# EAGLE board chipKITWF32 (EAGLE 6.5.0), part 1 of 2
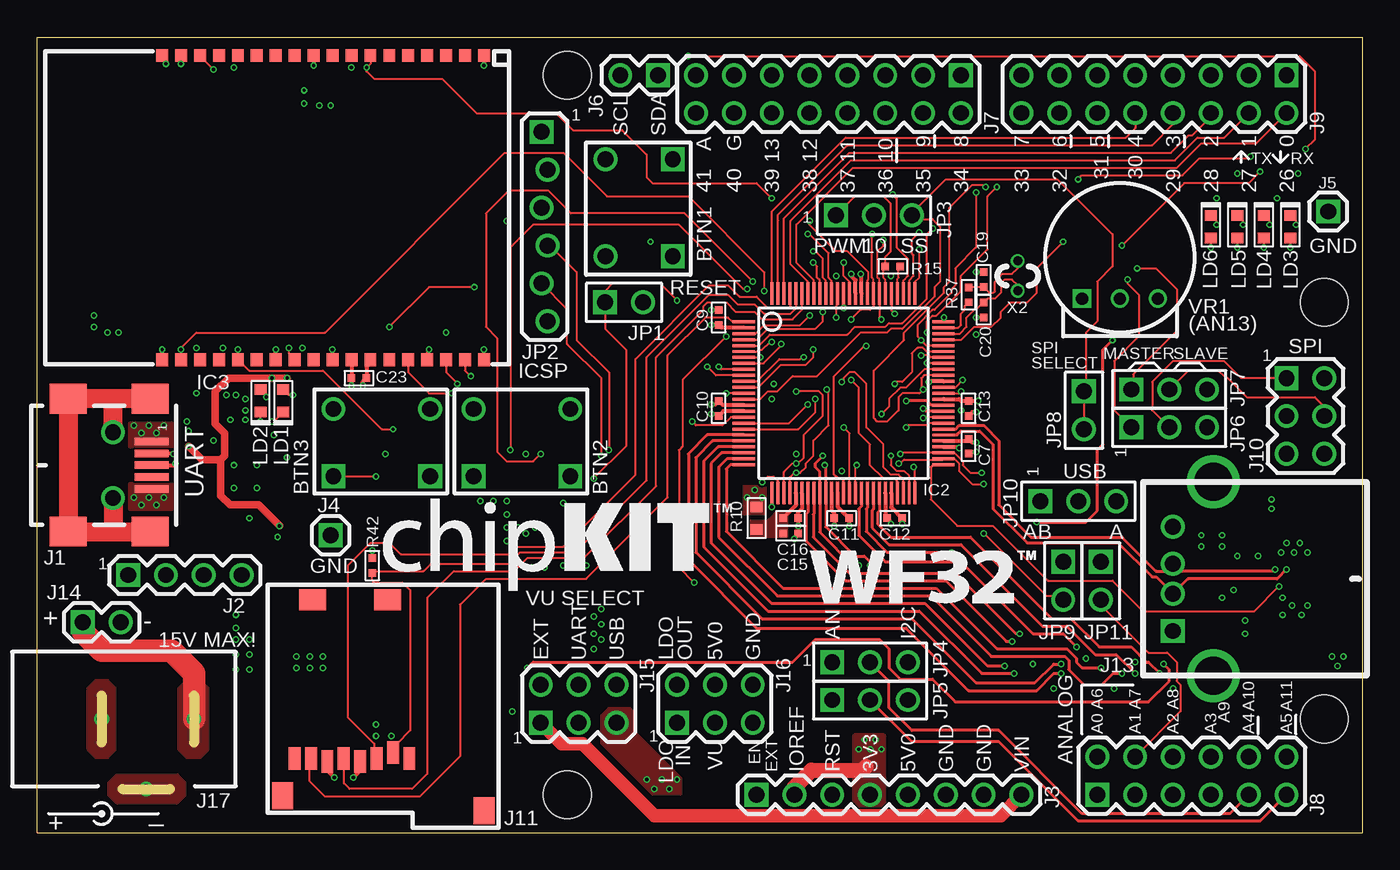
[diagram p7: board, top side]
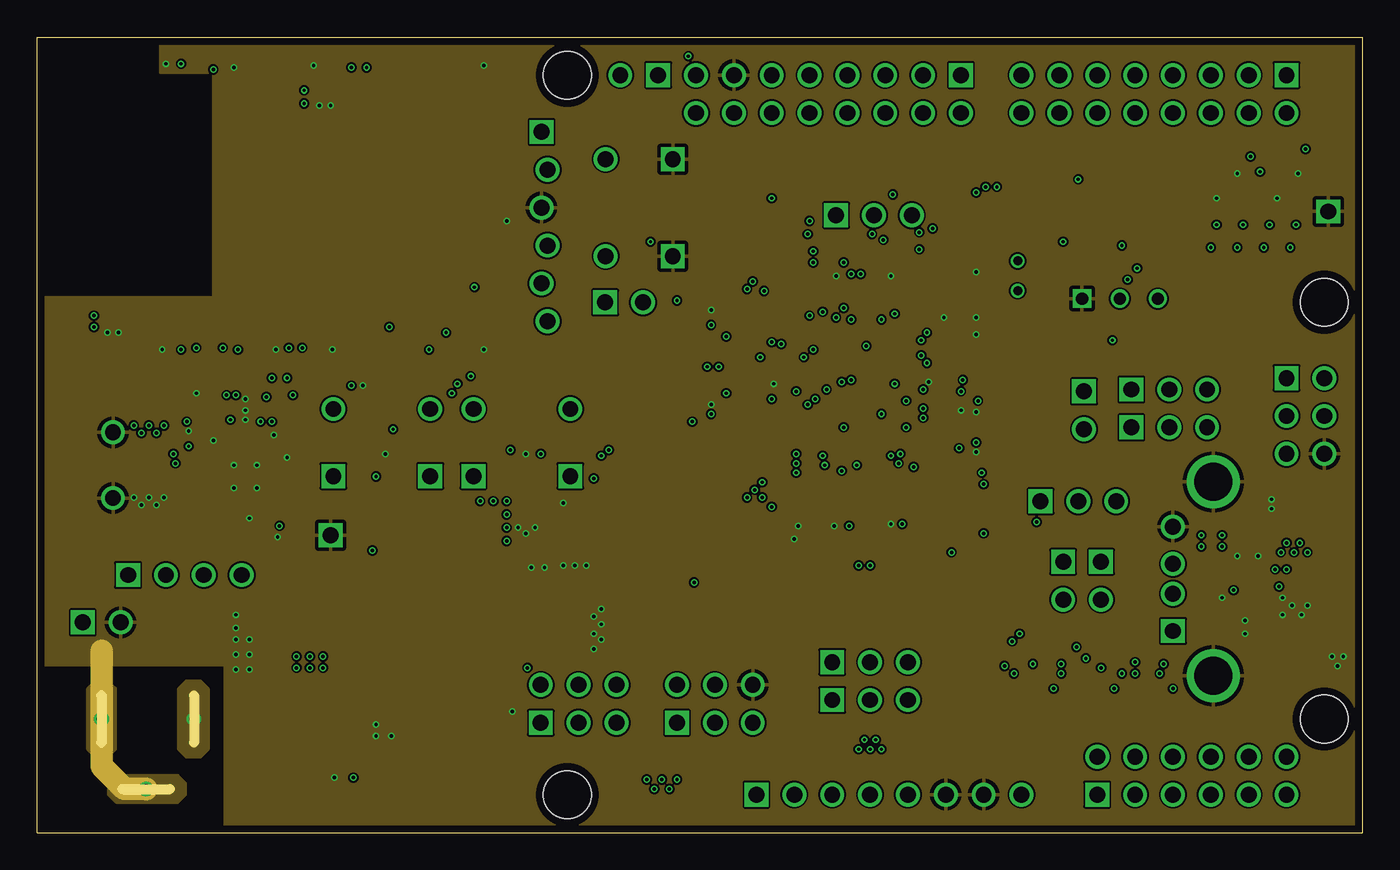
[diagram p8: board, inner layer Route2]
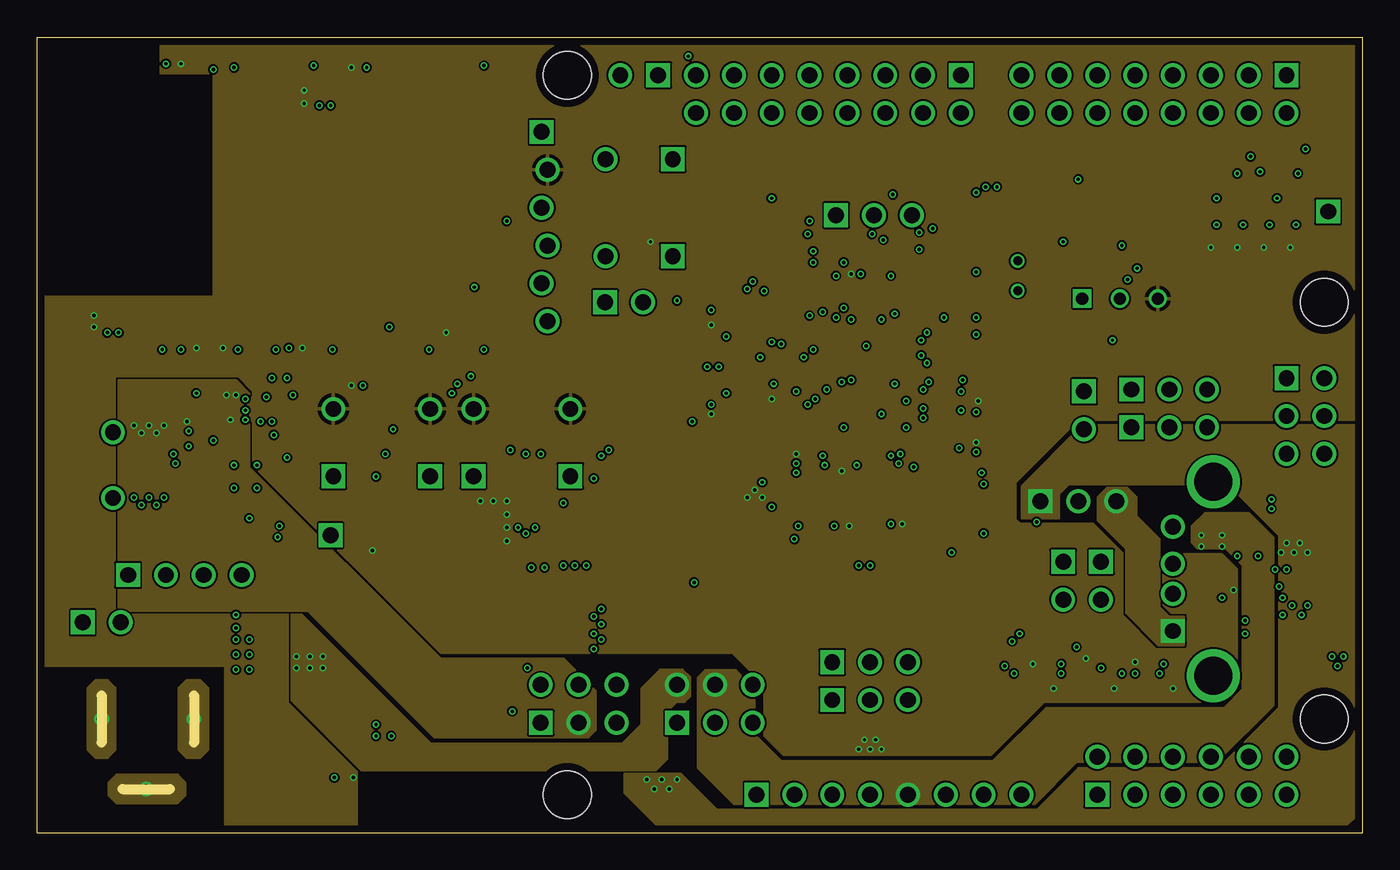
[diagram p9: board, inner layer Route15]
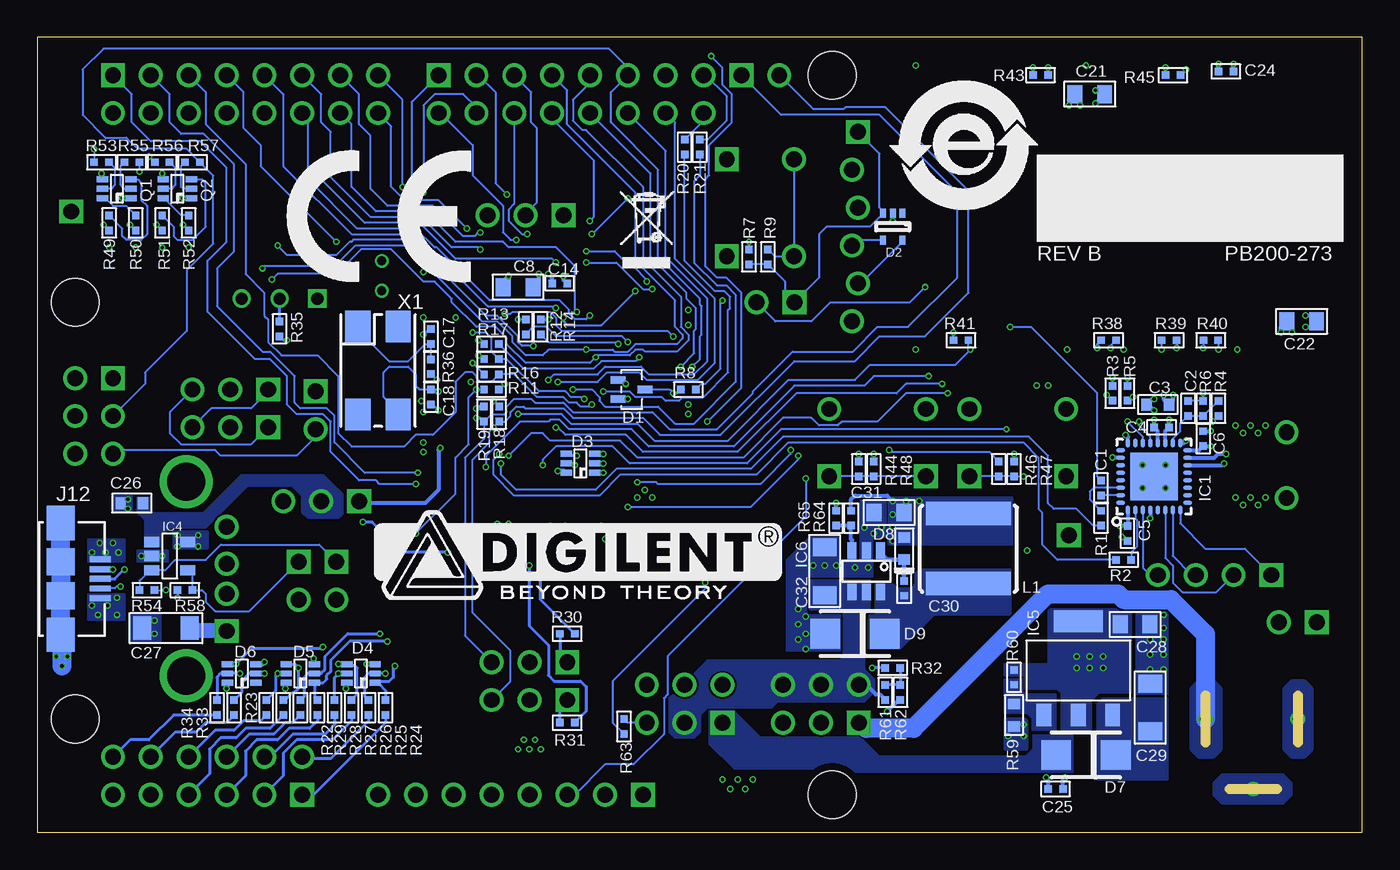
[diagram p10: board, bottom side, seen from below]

Size 88.9 x 53.34 mm. Coordinates in mm from the lower left corner, seen from the top.
Outline: 0,0 0,53.34 88.9,53.34 88.9,0 0,0
Copper layers ((1*2)+(15*16)): Top 0.035mm / dielectric 0.4mm / Route2 0.035mm / dielectric 0.6mm / Route15 0.035mm / dielectric 0.4mm / Bottom 0.035mm
Design rules "default *": minimum track width 5mil, minimum drill 9mil, track to track 5mil, track to pad 5mil, pad to pad 5mil, via to via 5mil, smd to smd 5mil, copper to edge 20mil, drill to drill 8mil, minimum pad ring 2mil, minimum via ring 2mil, stop-mask expansion 4mil, vias tented up to drill 15mil, thermal gap 10mil
Holes 3.2 mm at 35.56,50.8 86.36,35.56 86.36,7.62 35.56,2.54

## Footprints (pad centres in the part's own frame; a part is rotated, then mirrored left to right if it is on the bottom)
SW-P8008 = drill 1.067 square: 1A -2,3.5; 2A -2,-3 | drill 1.067: 1B 2.5,3.5; 2B 2.5,-3
C0402S = smd 0.5 x 0.5: 1 -0.5,0; 2 0.5,0
C0603S = smd 0.7 x 0.8: 1 -0.75,0; 2 0.75,0
C0805S = smd 1 x 1.2: 1 -1,0; 2 1,0
C1206S = smd 1.2 x 1.6: 1 -1.6,0; 2 1.6,0
SOT-323 = smd 0.5 x 1: 1 -0.65,-0.9; 2 0.65,-0.9; 3 0,0.9
SOT-323-5 = smd 0.4 x 0.6: 1 -0.65,-0.9; 2 0,-0.9; 3 0.65,-0.9; 4 0.65,0.9; 5 -0.65,0.9
SOT-363 = smd 0.4 x 0.762: 1 -0.635,-0.953; 2 0,-0.953; 3 0.635,-0.953; 4 0.635,0.953; 5 0,0.953; 6 -0.635,0.953
SMA = smd 2 x 2: A 2,0; C -2,0
D0603S = smd 0.7 x 0.8: A 0.75,0; C -0.75,0
QFN32 = smd 0.6 x 0.3: 1 -2.25,1.75; 2 -2.25,1.25; 3 -2.25,0.75; 4 -2.25,0.25; 5 -2.25,-0.25; 6 -2.25,-0.75; 7 -2.25,-1.25; 8 -2.25,-1.75; 17 2.25,-1.75; 18 2.25,-1.25; 19 2.25,-0.75; 20 2.25,-0.25; 21 2.25,0.25; 22 2.25,0.75; 23 2.25,1.25; 24 2.25,1.75 | smd 0.3 x 0.6: 9 -1.75,-2.25; 10 -1.25,-2.25; 11 -0.75,-2.25; 12 -0.25,-2.25; 13 0.25,-2.25; 14 0.75,-2.25; 15 1.25,-2.25; 16 1.75,-2.25; 25 1.75,2.25; 26 1.25,2.25; 27 0.75,2.25; 28 0.25,2.25; 29 -0.25,2.25; 30 -0.75,2.25; 31 -1.25,2.25; 32 -1.75,2.25 | smd 3.2 x 3.2: PAD 0,0
TQ100-PT = smd 1.5 x 0.2: 1 -6.7,4.8; 2 -6.7,4.4; 3 -6.7,4; 4 -6.7,3.6; 5 -6.7,3.2; 6 -6.7,2.8; 7 -6.7,2.4; 8 -6.7,2; 9 -6.7,1.6; 10 -6.7,1.2; 11 -6.7,0.8; 12 -6.7,0.4; 13 -6.7,0; 14 -6.7,-0.4; 15 -6.7,-0.8; 16 -6.7,-1.2; 17 -6.7,-1.6; 18 -6.7,-2; 19 -6.7,-2.4; 20 -6.7,-2.8; 21 -6.7,-3.2; 22 -6.7,-3.6; 23 -6.7,-4; 24 -6.7,-4.4; 25 -6.7,-4.8; 51 6.7,-4.8; 52 6.7,-4.4; 53 6.7,-4; 54 6.7,-3.6; 55 6.7,-3.2; 56 6.7,-2.8; 57 6.7,-2.4; 58 6.7,-2; 59 6.7,-1.6; 60 6.7,-1.2; 61 6.7,-0.8; 62 6.7,-0.4; 63 6.7,0; 64 6.7,0.4; 65 6.7,0.8; 66 6.7,1.2; 67 6.7,1.6; 68 6.7,2; 69 6.7,2.4; 70 6.7,2.8; 71 6.7,3.2; 72 6.7,3.6; 73 6.7,4; 74 6.7,4.4; 75 6.7,4.8 | smd 0.2 x 1.5: 26 -4.8,-6.7; 27 -4.4,-6.7; 28 -4,-6.7; 29 -3.6,-6.7; 30 -3.2,-6.7; 31 -2.8,-6.7; 32 -2.4,-6.7; 33 -2,-6.7; 34 -1.6,-6.7; 35 -1.2,-6.7; 36 -0.8,-6.7; 37 -0.4,-6.7; 38 0,-6.7; 39 0.4,-6.7; 40 0.8,-6.7; 41 1.2,-6.7; 42 1.6,-6.7; 43 2,-6.7; 44 2.4,-6.7; 45 2.8,-6.7; 46 3.2,-6.7; 47 3.6,-6.7; 48 4,-6.7; 49 4.4,-6.7; 50 4.8,-6.7; 76 4.8,6.7; 77 4.4,6.7; 78 4,6.7; 79 3.6,6.7; 80 3.2,6.7; 81 2.8,6.7; 82 2.4,6.7; 83 2,6.7; 84 1.6,6.7; 85 1.2,6.7; 86 0.8,6.7; 87 0.4,6.7; 88 0,6.7; 89 -0.4,6.7; 90 -0.8,6.7; 91 -1.2,6.7; 92 -1.6,6.7; 93 -2,6.7; 94 -2.4,6.7; 95 -2.8,6.7; 96 -3.2,6.7; 97 -3.6,6.7; 98 -4,6.7; 99 -4.4,6.7; 100 -4.8,6.7
MRF24WB0MA = smd 0.85 x 0.8: 1 -10.2,11.43; 2 -10.2,10.16; 3 -10.2,8.89; 4 -10.2,7.62; 5 -10.2,6.35; 6 -10.2,5.08; 7 -10.2,3.81; 8 -10.2,2.54; 9 -10.2,1.27; 10 -10.2,0; 11 -10.2,-1.27; 12 -10.2,-2.54; 13 -10.2,-3.81; 14 -10.2,-5.08; 15 -10.2,-6.35; 16 -10.2,-7.62; 17 -10.2,-8.89; 18 -10.2,-10.16; 19 10.2,-10.16; 20 10.2,-8.89; 21 10.2,-7.62; 22 10.2,-6.35; 23 10.2,-5.08; 24 10.2,-3.81; 25 10.2,-2.54; 26 10.2,-1.27; 27 10.2,0; 28 10.2,1.27; 29 10.2,2.54; 30 10.2,3.81; 31 10.2,5.08; 32 10.2,6.35; 33 10.2,7.62; 34 10.2,8.89; 35 10.2,10.16; 36 10.2,11.43
SOT23-5 = smd 0.7 x 1: 1 -0.95,-1.2; 2 0,-1.2; 3 0.95,-1.2; 4 0.95,1.2; 5 -0.95,1.2
SOT223 = smd 1 x 1.5: 1 -2.3,0; 2 0,0; 3 2.3,0 | smd 3.3 x 1.5: TAB 0,6.3
SOT23-6-CH = smd 0.6 x 1.1: 1 -0.95,-1.4; 2 0,-1.4; 3 0.95,-1.4; 4 0.95,1.4; 5 0,1.4; 6 -0.95,1.4
USB-AB-MINI = smd 0.5 x 2.3: 1 -1.6,2.6; 2 -0.8,2.6; 3 0,2.6; 4 0.8,2.6; 5 1.6,2.6 | smd 2 x 2.5: S1 -4.45,2.5; S2 -4.45,-3; S3 4.45,-3; S4 4.45,2.5 | drill 1.067: S5 -2.2,0; S6 2.2,0
HDR-1X4 = drill 1.067 square: 1 0,3.81 | drill 1.067: 2 0,1.27; 3 0,-1.27; 4 0,-3.81
HDR-1X8 = drill 1.067 square: 1 0,8.89 | drill 1.067: 2 0,6.35; 3 0,3.81; 4 0,1.27; 5 0,-1.27; 6 0,-3.81; 7 0,-6.35; 8 0,-8.89
HDR-1X1 = drill 1.067 square: 1 0,0
HDR-1X2 = drill 1.067 square: 1 0,1.27 | drill 1.067: 2 0,-1.27
HDR-2X8 = drill 1.067 square: 1 -1.27,8.89 | drill 1.067: 2 1.27,8.89; 3 -1.27,6.35; 4 1.27,6.35; 5 -1.27,3.81; 6 1.27,3.81; 7 -1.27,1.27; 8 1.27,1.27; 9 -1.27,-1.27; 10 1.27,-1.27; 11 -1.27,-3.81; 12 1.27,-3.81; 13 -1.27,-6.35; 14 1.27,-6.35; 15 -1.27,-8.89; 16 1.27,-8.89
HDR-2X6 = drill 1.067 square: 1 -1.27,6.35 | drill 1.067: 2 1.27,6.35; 3 -1.27,3.81; 4 1.27,3.81; 5 -1.27,1.27; 6 1.27,1.27; 7 -1.27,-1.27; 8 1.27,-1.27; 9 -1.27,-3.81; 10 1.27,-3.81; 11 -1.27,-6.35; 12 1.27,-6.35
HDR-2X3 = drill 1.067 square: 1 -1.27,2.54 | drill 1.067: 2 1.27,2.54; 3 -1.27,0; 4 1.27,0; 5 -1.27,-2.54; 6 1.27,-2.54
2908-05WB-MG = smd 0.8 x 1.5: 1 -1.6,4.05; 2 -0.5,3.65; 3 0.6,4.05; 4 1.7,4.25; 5 2.8,4.05; 6 3.9,4.25; 7 5,4.05; 8 6.1,4.05 | smd 1.8 x 1.4: P$9 4.9,-6.6; P$10 -0.15,-6.6 | smd 1.4 x 1.8: P$11 -6.6,7.55; P$12 6.9,6.55
USB-AB-MICRO = smd 0.4 x 1.4: 1 -1.3,4.1; 2 -0.65,4.1; 3 0,4.1; 4 0.65,4.1; 5 1.3,4.1 | smd 1.8 x 1.9: S1 -1.15,1.45; S2 1.14,1.45 | smd 2.3 x 1.9: S3 -3.75,1.45; S4 3.75,1.45
USB-A = drill 1.067 square: 1 -3.5,0 | drill 1.067: 2 -1,0; 3 1,0; 4 3.5,0 | drill 2.54: S1 -6.5,-2.71; S2 6.5,-2.71
KLD-0202S = drill 0.66: 1 6.2,0; 2 0,0; 3 3,-4.7
JPR-1X2 = drill 1.067 square: 1 0,1.27 | drill 1.067: 2 0,-1.27
HDR-1X6_OFFSET = drill 1.067 square: 1 -0.203,6.35 | drill 1.067: 2 0.203,3.81; 3 -0.203,1.27; 4 0.203,-1.27; 5 -0.203,-3.81; 6 0.203,-6.35
JPR-1X3 = drill 1.067 square: 1 0,2.54 | drill 1.067: 2 0,0; 3 0,-2.54
NR60XX = smd 1.6 x 5.7: 1 -2.35,0; 2 2.35,0
R0402S = smd 0.5 x 0.5: 1 -0.5,0; 2 0.5,0
R0603S = smd 0.7 x 0.8: 1 -0.75,0; 2 0.75,0
BOURNS-3352T = drill 0.813 square: 1 -2.54,0 | drill 0.813: 2 0,0; 3 2.54,0
FQ7050B = smd 2.1 x 1.7: 1 -2.95,-1.35; 2 2.95,-1.35; 3 2.95,1.35; 4 -2.95,1.35
XT-T38 = drill 0.61: 1 -1,0; 2 1,0

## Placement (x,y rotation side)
BTN1  SW-P8008  [SW-P8008]  40.64,42.16 180 top
BTN2  SW-P8008  [SW-P8008]  32.77,25.91 90 top
BTN3  SW-P8008  [SW-P8008]  23.37,25.91 90 top
C1  0.1uF  [C0402S]  17.53,23.11 90 bottom
C2  0.1uF  [C0402S]  11.68,28.45 90 bottom
C3  4.7uF  [C0603S]  13.72,28.7 180 bottom
C4  0.1uF  [C0402S]  13.46,27.18 180 bottom
C5  0.1uF  [C0402S]  15.75,20.07 270 bottom
C6  0.1uF  [C0402S]  10.67,26.42 90 bottom
C7  0.1uF  [C0402S]  62.48,25.91 270 top
C8  10uF/10V  [C0805S]  56.64,36.58 180 bottom
C9  0.1uF  [C0402S]  45.72,34.54 90 top
C10  0.1uF  [C0402S]  45.72,28.45 90 top
C11  0.1uF  [C0402S]  53.98,21.08 180 top
C12  0.1uF  [C0402S]  57.53,21.08 180 top
C13  0.1uF  [C0402S]  62.48,28.45 270 top
C14  0.1uF  [C0402S]  53.85,36.83 0 bottom
C15  1uF  [C0402S]  50.55,20.07 0 top
C16  0.1uF  [C0402S]  50.55,21.08 0 top
C17  30pF  [C0402S]  62.48,33.27 90 bottom
C18  30pF  [C0402S]  62.48,29.21 270 bottom
C19  30pF  [C0402S]  63.5,37.08 90 top
C20  30pF  [C0402S]  63.5,35.05 270 top
C21  10uF  [C0805S]  18.29,49.53 180 bottom
C22  10uF  [C0805S]  4.06,34.29 180 bottom
C23  0.1uF  [C0402S]  21.59,30.48 0 top
C24  0.1uF  [C0402S]  9.14,51.05 0 bottom
C25  0.1uF  [C0402S]  20.57,2.92 0 bottom
C26  6.8uF/10V  [C0603S]  82.55,22.1 180 bottom
C27  100uF/10V  [C1206S]  80.26,13.72 180 bottom
C28  10uF/10V  [C0805S]  15.24,13.97 0 bottom
C29  10uF/25V  [C1206S]  14.22,8.38 90 bottom
C30  100nF  [C0402S]  30.73,16.38 270 bottom
C31  10uF  [C0805S]  31.75,21.46 180 bottom
C32  10uF/25V  [C1206S]  36.07,17.53 90 bottom
D1  BAV99W  [SOT-323]  49.02,29.72 270 bottom
D2  NSQA6V8  [SOT-323-5]  31.5,40.64 180 bottom
D3  BAV70S  [SOT-363]  52.45,24.77 90 bottom
D4  BAV70S  [SOT-363]  67.18,10.67 90 bottom
D5  BAV70S  [SOT-363]  71.25,10.67 90 bottom
D6  BAV70S  [SOT-363]  75.18,10.67 90 bottom
D7  B240A-13-F  [SMA]  18.54,5.21 180 bottom
D8  CDSU4148  [D0603S]  30.73,19.05 90 bottom
D9  B240A-13-F  [SMA]  34.04,13.34 180 bottom
IC1  FT232RQ  [QFN32]  13.97,23.88 90 bottom
IC2  PIC32MX695F512L-80I/PT  [TQ100-PT]  54.1,29.46 0 top
IC3  MRF24WG0MA  [MRF24WB0MA]  18.54,41.91 270 top
IC4  TPS2051BDBVR  [SOT23-5]  80.01,18.54 270 bottom
IC5  NCP1117DT50T3G  [SOT223]  19.05,7.87 0 bottom
IC6  MCP16301T-I/CHY  [SOT23-6-CH]  33.27,17.53 180 bottom
J1  USB-AB-MINI  [USB-AB-MINI]  5.08,24.64 270 top
J2  No Load  [HDR-1X4]  9.91,17.27 90 top
J3  ST. Female  [HDR-1X8]  57.15,2.54 90 top
J4  ST. Male  [HDR-1X1]  19.68,19.94 0 top
J5  ST. Male  [HDR-1X1]  86.61,41.66 90 top
J6  ST. Female  [HDR-1X2]  40.39,50.8 270 top
J7  ST. Female  [HDR-2X8]  53.09,49.53 270 top
J8  ST. Female  [HDR-2X6]  77.47,3.81 90 top
J9  ST. Female  [HDR-2X8]  74.93,49.53 270 top
J10  ST. Male  [HDR-2X3]  85.09,27.94 0 top
J11  2908-05WB-MG  [2908-05WB-MG]  23.37,9.02 180 top
J12  USB-AB-MICRO  [USB-AB-MICRO]  88.77,17.02 270 bottom
J13  USB-A  [USB-A]  76.2,17.02 90 top
J14  ST. Male  [HDR-1X2]  4.32,14.1 90 top
J15  ST. Male  [HDR-2X3]  36.32,8.64 90 top
J16  ST. Male  [HDR-2X3]  45.47,8.64 90 top
J17  CON-COAX-KLD0202-S  [KLD-0202S]  4.32,7.62 0 top
JP1  ST. Male  [JPR-1X2]  39.37,35.56 90 top
JP2  No Load  [HDR-1X6_OFFSET]  34.04,40.64 0 top
JP3  JPR-1X3  [JPR-1X3]  56.13,41.4 90 top
JP4  ST. Male  [JPR-1X3]  55.88,11.43 90 top
JP5  ST. Male  [JPR-1X3]  55.88,8.89 90 top
JP6  JPR-1X3  [JPR-1X3]  75.95,27.18 90 top
JP7  JPR-1X3  [JPR-1X3]  75.95,29.72 90 top
JP8  No Load  [JPR-1X2]  70.23,28.32 0 top
JP9  ST. Male  [JPR-1X2]  68.83,16.89 0 top
JP10  ST. Male  [JPR-1X3]  69.85,22.23 90 top
JP11  ST. Male  [JPR-1X2]  71.37,16.89 0 top
L1  NR6028T150M  [NR60XX]  26.42,19.05 90 bottom
LD1  Red  [D0603S]  16.51,28.96 90 top
LD2  Red  [D0603S]  14.99,28.96 90 top
LD3  Green  [D0603S]  84.07,40.64 270 top
LD4  Green  [D0603S]  82.3,40.64 270 top
LD5  Green  [D0603S]  80.52,40.64 270 top
LD6  Green  [D0603S]  78.74,40.64 270 top
LOGO1  DIGILENT_INC-BT-1000  [DIGILENT_BEYOND_1000_LOGO]  66.29,15.62 0 bottom
LOGO2  CE  [CE_LOGO]  72.39,36.83 0 bottom
LOGO3  CHIPKIT  [CHIPKIT_LOGO]  23.24,16.26 0 top
LOGO4  WEEE-S  [WEEE_LOGO]  49.28,37.08 0 bottom
LOGO5  ROHS-CHINA  [ROHS_CHINA_LOGO]  32.77,41.02 0 bottom
Q1  MBT3904DW1T1  [SOT-363]  83.57,43.18 90 bottom
Q2  MBT3904DW1T1  [SOT-363]  79.5,43.18 90 bottom
R1  2.2K  [R0402S]  17.53,21.08 270 bottom
R2  1K  [R0402S]  16,18.29 180 bottom
R3  470  [R0402S]  16.76,29.46 90 bottom
R4  4.7K  [R0402S]  9.65,28.45 270 bottom
R5  470  [R0402S]  15.75,29.46 90 bottom
R6  10K  [R0402S]  10.67,28.45 270 bottom
R7  10K  [R0402S]  41.15,38.61 90 bottom
R8  50  [R0402S]  45.21,29.72 0 bottom
R9  200  [R0402S]  39.88,38.61 270 bottom
R10  0  [R0603S]  48.26,21.08 270 top
R11  1K  [R0402S]  58.42,29.72 180 bottom
R12  1K  [R0402S]  56.13,33.91 90 bottom
R13  1K  [R0402S]  58.42,32.77 180 bottom
R14  1K  [R0402S]  55.12,33.91 90 bottom
R15  1K  [R0402S]  57.4,37.97 180 top
R16  1K  [R0402S]  58.42,30.73 0 bottom
R17  1K  [R0402S]  58.42,31.75 0 bottom
R18  2.2K  [R0402S]  57.91,28.07 270 bottom
R19  2.2K  [R0402S]  58.93,28.07 270 bottom
R20  200  [R0402S]  45.47,45.97 90 bottom
R21  200  [R0402S]  44.45,45.97 90 bottom
R22  200  [R0402S]  72.39,8.38 270 bottom
R23  200  [R0402S]  73.53,8.38 270 bottom
R24  200  [R0402S]  65.53,8.38 270 bottom
R25  200  [R0402S]  66.67,8.38 270 bottom
R26  200  [R0402S]  67.82,8.38 270 bottom
R27  200  [R0402S]  68.96,8.38 270 bottom
R28  200  [R0402S]  70.1,8.38 270 bottom
R29  200  [R0402S]  71.25,8.38 270 bottom
R30  200  [R0402S]  53.34,13.34 180 bottom
R31  200  [R0402S]  53.34,7.37 180 bottom
R32  200  [R0402S]  31.5,11.05 0 bottom
R33  200  [R0402S]  75.69,8.38 270 bottom
R34  200  [R0402S]  76.83,8.38 270 bottom
R35  1K  [R0402S]  72.64,33.78 90 bottom
R36  680  [R0402S]  62.48,31.24 270 bottom
R37  0  [R0402S]  62.48,36.07 270 top
R38  4.7K  [R0402S]  17.02,33.02 180 bottom
R39  10K  [R0402S]  12.95,33.02 0 bottom
R40  10K  [R0402S]  10.16,33.02 180 bottom
R41  10K  [R0402S]  26.92,33.02 180 bottom
R42  10K  [R0402S]  22.48,17.91 90 top
R43  10K  [R0402S]  21.59,50.8 0 bottom
R44  10K  [R0402S]  33.78,24.38 270 bottom
R45  10K  [R0402S]  12.7,50.8 0 bottom
R46  10K  [R0402S]  24.38,24.38 270 bottom
R47  10K  [R0402S]  23.37,24.38 270 bottom
R48  10K  [R0402S]  32.77,24.38 270 bottom
R49  470  [R0402S]  84.07,40.89 270 bottom
R50  470  [R0402S]  82.3,40.89 270 bottom
R51  470  [R0402S]  80.52,40.89 270 bottom
R52  470  [R0402S]  78.74,40.89 270 bottom
R53  4.7K  [R0402S]  84.58,44.96 0 bottom
R54  10K  [R0402S]  81.53,16.26 0 bottom
R55  4.7K  [R0402S]  82.55,44.96 180 bottom
R56  4.7K  [R0402S]  80.52,44.96 0 bottom
R57  4.7K  [R0402S]  78.49,44.96 180 bottom
R58  10K  [R0402S]  78.99,16.26 0 bottom
R59  0  [R0603S]  23.37,7.87 90 bottom
R60  NL  [R0402S]  23.37,10.41 90 bottom
R61  10K  [R0402S]  32,9.4 270 bottom
R62  1K  [R0402S]  30.99,9.4 90 bottom
R63  1K  [R0402S]  49.53,7.11 90 bottom
R64  31.2K  [R0402S]  34.29,21.08 90 bottom
R65  10K  [R0402S]  35.31,21.08 270 bottom
U$1  CHIPKIT_WF32_LOGO  [CHIPKIT_WF32_LOGO]  51.82,15.37 0 top
VR1  10K  [BOURNS-3352T]  72.64,35.81 0 top
X1  FQ7050B-8.000  [FQ7050B]  66.04,30.99 270 bottom
X2  No Load  [XT-T38]  65.79,37.34 270 top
